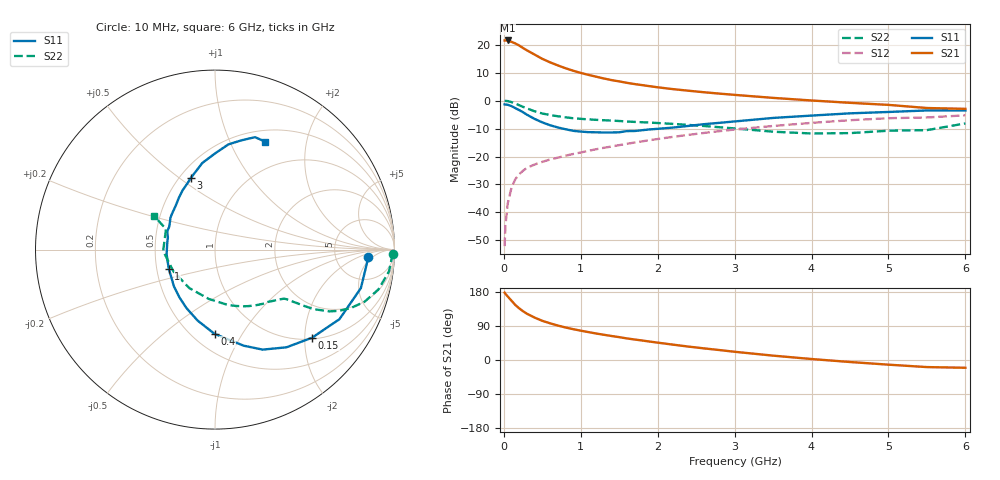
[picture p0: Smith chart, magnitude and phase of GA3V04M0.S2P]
! Infineon Technologies  Discrete & RF Semiconductors
! BF775
! Si NPN RF Bipolar Junction Transistor in SOT23
! VCE = 3 V  IC = 4 mA
! Common Emitter S-Parameters:  May  1996
# GHz  S  MA  R  50
!  f  S11  S21  S12  S22
! GHz  MAG  ANG  MAG  ANG  MAG  ANG  MAG  ANG
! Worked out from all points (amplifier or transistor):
!   36 points, 10 MHz to 6 GHz, reference 50 ohm
!   highest |S21| = 21.5 dB at 50 MHz (marker M1)
!   |S21| within 3 dB of that: start of sweep to 267.9 MHz
!   unconditionally stable (mu >= 1): 871 MHz to 3.578 GHz
!   at 250 MHz: K = 0.43, MSG = 21.9 dB, |S12| = -25.1 dB
!   at 1.4 GHz: K = 1.13, MAG = 9.7 dB, |S12| = -16.4 dB
!   at 6 GHz: K = 0.97, MSG = 1.2 dB, |S12| = -5.3 dB
!   S11 on the Smith chart (normalised r, x): 10 MHz: 12, -4; 150 MHz: 1.03, -2.17; 400 MHz: 0.64, -0.77; 1 GHz: 0.58, -0.14; 3 GHz: 0.57, +0.56; 6 GHz: 0.64, +1.37
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0.01  0.8546 -2.9  11.8 177.7  0.0025 89.0  0.9934 -1.3
0.02  0.8483 -5.9  11.81 174.8  0.0057 85.4  0.9861 -2.8
0.05  0.8406 -14.8  11.84 167.7  0.0144 80.7  0.9767 -7.2
0.1  0.7944 -29.2  11.18 156.4  0.0279 74.8  0.9373 -13.7
0.15  0.7305 -42.2  10.45 145.0  0.0395 68.3  0.8827 -19.2
0.2  0.6745 -53.8  9.609 136.3  0.0484 63.5  0.8238 -23.3
0.25  0.6174 -64.5  8.667 128.7  0.0558 59.5  0.7701 -26.3
0.3  0.5586 -73.4  7.891 122.1  0.0626 57.6  0.7237 -28.4
0.4  0.4695 -90.3  6.622 111.9  0.0719 54.5  0.6425 -31.1
0.5  0.407 -103.8  5.555 103.4  0.0802 53.3  0.5865 -32.3
0.6  0.3624 -116.1  4.818 96.9  0.0885 52.9  0.5516 -33.0
0.7  0.3309 -127.1  4.253 91.0  0.0952 52.8  0.5239 -33.7
0.8  0.3074 -138.0  3.784 85.9  0.1032 52.8  0.5018 -34.2
1  0.2788 -157.3  3.113 77.4  0.1179 54.0  0.4707 -35.5
1.1  0.2723 -165.5  2.873 73.6  0.1264 54.1  0.4608 -36.8
1.6  0.2845 159.3  2.07 56.9  0.1685 53.8  0.4225 -43.1
2.2  0.3286 131.7  1.598 40.5  0.2245 51.3  0.3827 -54.4
3  0.423 108.3  1.262 21.7  0.3032 44.2  0.3176 -76.6
3.5  0.4886 98.2  1.115 11.5  0.3512 38.5  0.2772 -97.1
4.5  0.5904 82.8  0.91 -5.3  0.4449 25.7  0.2618 -152.6
5.5  0.6649 70.4  0.735 -18.7  0.4985 10.6  0.296 157.2
6  0.6632 65.0  0.71 -20.5  0.5439 6.4  0.3899 151.0
